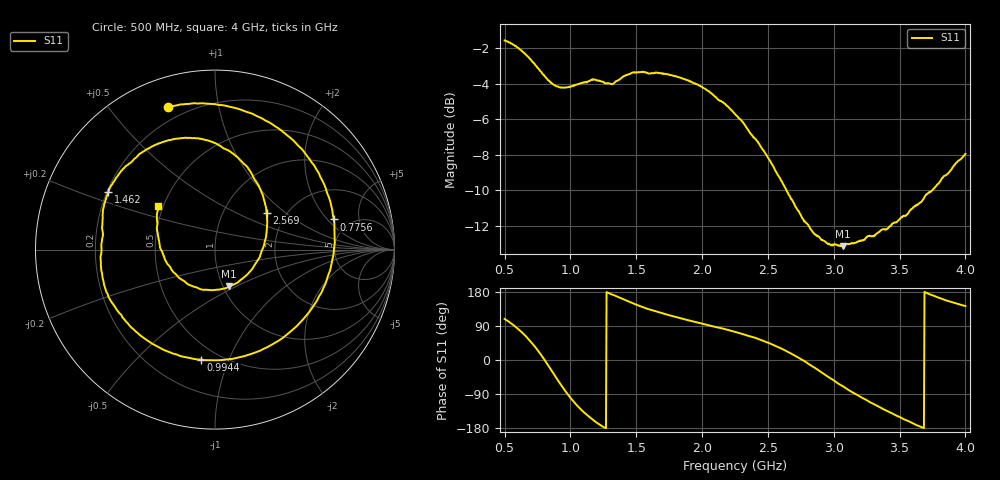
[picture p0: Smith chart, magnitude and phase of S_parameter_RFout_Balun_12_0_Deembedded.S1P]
!Agilent Technologies,E5071B,MY42403504,A.06.51
!Date: Wed Feb 26 14:57:41 2014
!Data & Calibration Information:
!Freq	S11:SOLT1(ON)
# Hz S dB R 50
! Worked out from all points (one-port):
!   801 points, 500 MHz to 4 GHz, reference 50 ohm
!   lowest |S11| = -13.2 dB at 3.068 GHz (marker M1), VSWR 1.56, Z = 53.4 - j23 ohm
!   |S11| at or under -10 dB: 2.64 GHz to 3.75 GHz (1.11 GHz wide, 34.7 % of centre)
!   S11 on the Smith chart (normalised r, x): 500 MHz: 0.14, +0.71; 775.6 MHz: 3.74, +2.36; 994.4 MHz: 0.40, -0.80; 1.462 GHz: 0.21, +0.24; 2.569 GHz: 1.60, +0.74; 4 GHz: 0.47, +0.27
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5e8  -1.55 108.3
5.7875e8  -1.87 88.8
6.44375e8  -2.25 68.7
7.1e8  -2.74 43.8
7.75625e8  -3.31 14.3
8.10625e8  -3.62 -3.4
8.5e8  -3.94 -24.3
8.9375e8  -4.14 -47.7
9.375e8  -4.22 -70.3
9.94375e8  -4.19 -97.2
1.0775e9  -3.98 -129.7
1.165e9  -3.75 -156.2
1.2525e9  -3.90 -176.9
1.375e9  -3.75 164.4
1.4625e9  -3.40 151.4
1.655e9  -3.37 127.7
1.8125e9  -3.62 112.3
2.01375e9  -4.25 94.9
2.25e9  -5.71 74.1
2.569375e9  -9.06 35.3
2.6875e9  -10.60 14.8
2.85375e9  -12.46 -20.2
3.068125e9  -13.16 -69.1
3.125e9  -13.03 -81.9
3.34375e9  -12.37 -123.5
3.5625e9  -11.34 -160.7
3.71125e9  -10.22 175.8
4e9  -7.96 142.6
